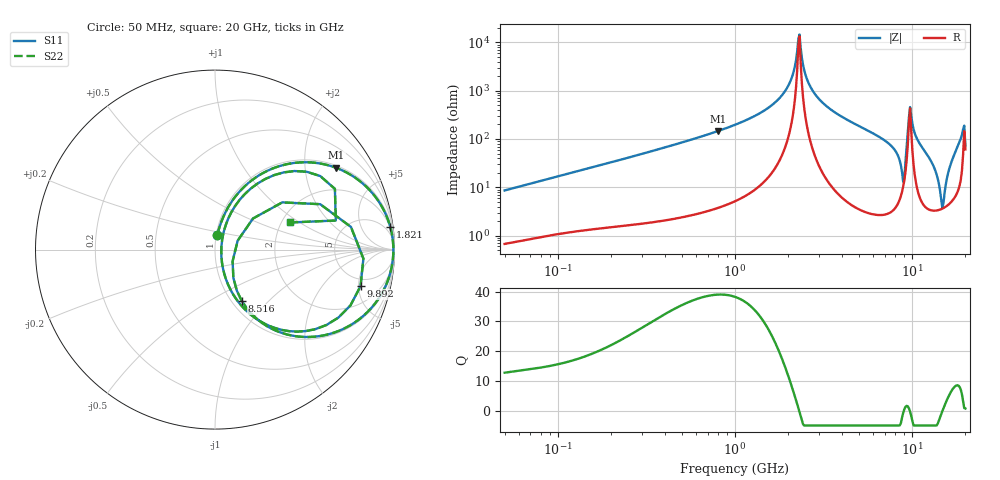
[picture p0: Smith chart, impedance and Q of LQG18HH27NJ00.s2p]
!Murata Part Number: LQG18HH27NJ00
!These Parameters are Measured in Series Mode Connection
!  o--[Z]--o
!Port1  Port2
!  o-------o
!Freq. Start=50[MHz] Stop=20[GHz], 401[Steps]
# Hz S RI R 50
!Freq.(Hz) S11(Real) S11(Imag) S21(Real) S21(Imag) S12(Real) S12(Imag) S22(Real) S22(Imag)
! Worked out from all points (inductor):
!   401 points, 50 MHz to 20 GHz, reference 50 ohm
!   read as one part in series: L = 27.1 nH near 51.52 MHz
!   highest Q = 39 at 798.8 MHz (marker M1), where L = 29 nH
!   self-resonance near 2.279 GHz
!   S11 on the Smith chart (normalised r, x): 50 MHz: 1.01, +0.17; 1.821 GHz: 2, +15; 8.516 GHz: 1.11, -0.71; 9.892 GHz: 3.91, -5.28; 20 GHz: 2.22, +0.84
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5e7  0.0139 0.0841  0.9861 -0.0841  0.9861 -0.0841  0.0139 0.0841
1.364002e8  0.0595 0.2101  0.9405 -0.2101  0.9405 -0.2101  0.0595 0.2101
3.721004e8  0.283 0.4347  0.717 -0.4347  0.717 -0.4347  0.283 0.4347
7.987718e8  0.6753 0.4556  0.3247 -0.4556  0.3247 -0.4556  0.6753 0.4556
1e9  0.7889 0.3952  0.2111 -0.3952  0.2111 -0.3952  0.7889 0.3952
1.820564e9  0.9765 0.1267  0.0235 -0.1267  0.0235 -0.1267  0.9765 0.1267
2.083303e9  0.9905 0.0546  0.00955 -0.0546  0.00955 -0.0546  0.9905 0.0546
2.313601e9  0.9938 -0.00271  0.00624 0.00271  0.00624 0.00271  0.9938 -0.00271
2.493527e9  0.9919 -0.0441  0.00807 0.0441  0.00807 0.0441  0.9919 -0.0441
2.728004e9  0.985 -0.0941  0.015 0.0941  0.015 0.0941  0.985 -0.0941
3.850025e9  0.9043 -0.2832  0.0957 0.2832  0.0957 0.2832  0.9043 -0.2832
7.442007e9  0.386 -0.4685  0.614 0.4685  0.614 0.4685  0.386 -0.4685
8.516016e9  0.1488 -0.2854  0.8512 0.2854  0.8512 0.2854  0.1488 -0.2854
8.907419e9  0.0982 -0.0647  0.9018 0.0647  0.9018 0.0647  0.0982 -0.0647
9.316812e9  0.3746 0.263  0.6254 -0.263  0.6254 -0.263  0.3746 0.263
9.892087e9  0.8111 -0.2031  0.1889 0.2031  0.1889 0.2031  0.8111 -0.2031
1.066139e10  0.5051 -0.454  0.4949 0.454  0.4949 0.454  0.5051 -0.454
1.295331e10  0.116 -0.2723  0.884 0.2723  0.884 0.2723  0.116 -0.2723
1.482269e10  0.035 -0.00622  0.965 0.00622  0.965 0.00622  0.035 -0.00622
1.721783e10  0.2002 0.3408  0.7998 -0.3408  0.7998 -0.3408  0.2002 0.3408
1.855685e10  0.4425 0.4378  0.5575 -0.4378  0.5575 -0.4378  0.4425 0.4378
2e10  0.4184 0.1511  0.5816 -0.1511  0.5816 -0.1511  0.4184 0.1511
